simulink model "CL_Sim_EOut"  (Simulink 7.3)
settings: Solver=ode3  StartTime=0.0  StopTime=32  FixedStep=0.02  RelTol=1e-3
InitFcn:
  | [np,n]=size(time);
  | tfin= time(np);
  | Xini= xx(np,:);
  | Xfini= xfc(np,:);
  | dyin= dy(np,:);
  | dzin= dz(np,:);
  | Thin= Dthrust(np,:);
StopFcn:
  | Pl2
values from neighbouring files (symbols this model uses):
  Afc = [    [fcs.m]
  Bfc = [    [fcs.m]
  Cfc = [    [fcs.m]
  d2r = pi/180    (= 0.0174532925199)    [run.m]
  Dfc = [    [fcs.m]
  LBThrust = 0.96097e+6    (= 960970)    [run.m]
undefined symbols (not defined in the file or in its folder): Av2, Bv2, Cv2, Dv2, ThVC_eo

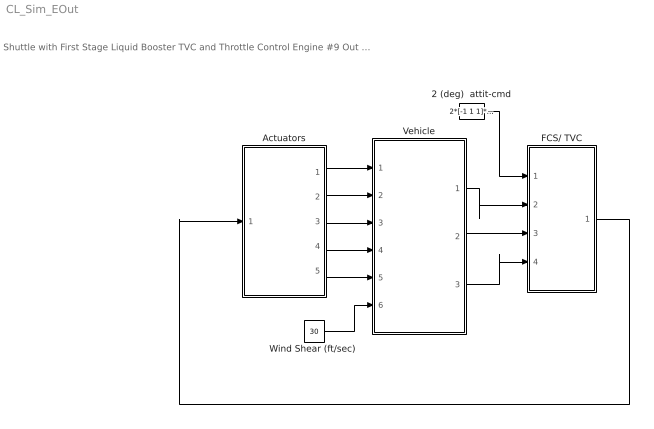
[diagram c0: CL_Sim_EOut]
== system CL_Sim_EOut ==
  note: Shuttle with First Stage Liquid Booster TVC and Throttle Control Engine #9 Out Simulation
  2 (deg)  attit-cmd : Constant  Value=2*[-1 1 1]*d2r  OutDataType=sfix(16)  OutScaling=2^0
  Actuators : Subsystem
  FCS/ TVC : Subsystem
  Vehicle : Subsystem
  "Wind Shear (ft/sec) " : Constant  Value=30  OutDataType=sfix(16)  OutScaling=2^0
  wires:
  FCS/ TVC/1(TVC) -> Actuators/1(TVC)
  Vehicle/1(atti) -> FCS/ TVC/2(atti)
  Vehicle/2(rate) -> FCS/ TVC/3(rate)
  Vehicle/3(accel) -> FCS/ TVC/4(accel)
  "Wind Shear (ft/sec) "/1 -> Vehicle/6(Gust)
  2 (deg)  attit-cmd/1 -> FCS/ TVC/1(atti-cmd)
  Actuators/1(dy (pitch)) -> Vehicle/1(dy)
  Actuators/5(DThrottle) -> Vehicle/5(Dthro)
  Actuators/4(dzdd) -> Vehicle/4(dzdd)
  Actuators/3(dz (yaw)) -> Vehicle/3(dz)
  Actuators/2(dydd) -> Vehicle/2(dydd)

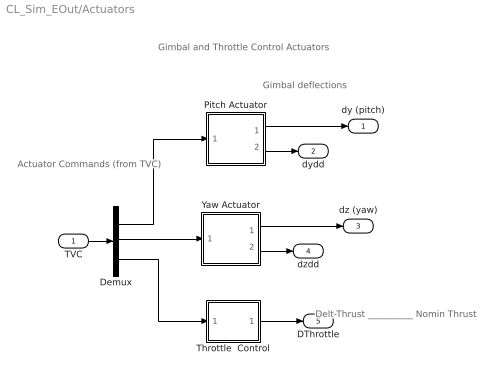
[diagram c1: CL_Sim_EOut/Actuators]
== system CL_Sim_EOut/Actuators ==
  note: Gimbal and Throttle Control Actuators
  note: Actuator Commands (from TVC)
  note: Gimbal deflections
  note: Delt-Thrust __________ Nomin Thrust
  TVC : Inport  OutDataType=sfix(16)  OutScaling=2^0
  Demux : Demux  Outputs=[9, 9, 6]
  Pitch Actuator : Subsystem
  Throttle  Control : Subsystem
  Yaw Actuator : Subsystem
  dy (pitch) : Outport  OutDataType=sfix(16)  OutScaling=2^0
  dydd : Outport  Port=2  OutDataType=sfix(16)  OutScaling=2^0
  dz (yaw) : Outport  Port=3  OutDataType=sfix(16)  OutScaling=2^0
  dzdd : Outport  Port=4  OutDataType=sfix(16)  OutScaling=2^0
  DThrottle : Outport  Port=5  OutDataType=sfix(16)  OutScaling=2^0
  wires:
  Demux/3 -> Throttle  Control/1(thi)
  Demux/1 -> Pitch Actuator/1(dy-c)
  Demux/2 -> Yaw Actuator/1(dz-c)
  Pitch Actuator/1(dy) -> dy (pitch)/1
  TVC/1 -> Demux/1
  Throttle  Control/1(tho) -> DThrottle/1
  Yaw Actuator/1(dz) -> dz (yaw)/1
  Pitch Actuator/2(dydd) -> dydd/1
  Yaw Actuator/2(dzdd) -> dzdd/1

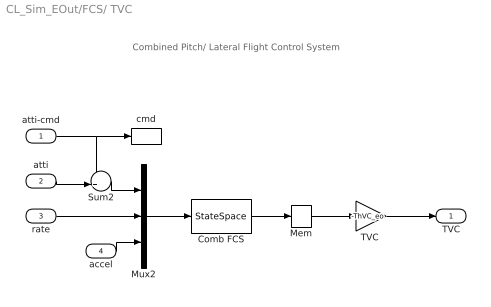
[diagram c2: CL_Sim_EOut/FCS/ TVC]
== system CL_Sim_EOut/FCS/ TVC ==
  note: Combined Pitch/ Lateral Flight Control System
  atti-cmd : Inport  OutDataType=sfix(16)  OutScaling=2^0
  atti : Inport  Port=2  OutDataType=sfix(16)  OutScaling=2^0
  rate : Inport  Port=3  OutDataType=sfix(16)  OutScaling=2^0
  accel : Inport  Port=4  OutDataType=sfix(16)  OutScaling=2^0
  Comb FCS : StateSpace  A=Afc  B=Bfc  C=Cfc  D=Dfc  X0=Xfini
  Mem : Memory
  Mux2 : Mux  Inputs=[3, 3, 2]
  Sum2 : Sum  Inputs=-+|  OutDataType=sfix(16)  OutScaling=2^0
  "TVC " : Gain  Gain=-ThVC_eo  Multiplication=Matrix(K*u) (u vector)  ParameterDataType=sfix(16)  ParameterScaling=2^0  OutDataType=sfix(16)  OutScaling=2^0
  cmd : ToWorkspace  VariableName=cmd2  SampleTime=-1  SaveFormat=Array
  TVC : Outport  OutDataType=sfix(16)  OutScaling=2^0
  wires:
  Mux2/1 -> Comb FCS/1
  accel/1 -> Mux2/3
  rate/1 -> Mux2/2
  "TVC "/1 -> TVC/1
  Sum2/1 -> Mux2/1
  atti/1 -> Sum2/2
  atti-cmd/1 -> Sum2/1, cmd/1
  Mem/1 -> "TVC "/1
  Comb FCS/1 -> Mem/1

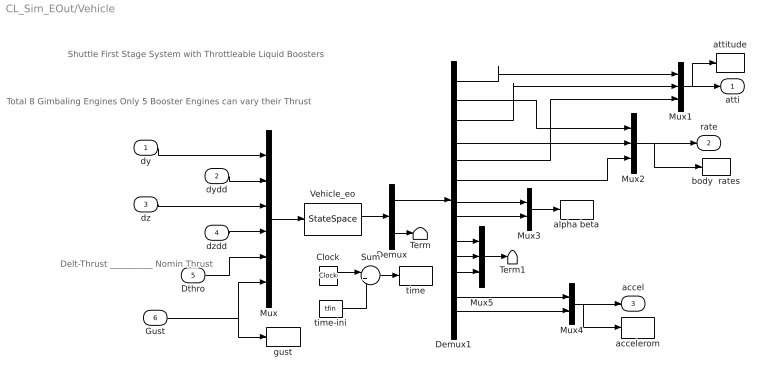
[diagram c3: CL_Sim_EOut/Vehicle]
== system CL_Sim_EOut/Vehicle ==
  note: Shuttle First Stage System with Throttleable Liquid Boosters
  note: Total 8 Gimbaling Engines Only 5 Booster Engines can vary their Thrust
  note: Delt-Thrust __________ Nomin Thrust
  dy : Inport  OutDataType=sfix(16)  OutScaling=2^0
  dydd : Inport  Port=2  OutDataType=sfix(16)  OutScaling=2^0
  dz : Inport  Port=3  OutDataType=sfix(16)  OutScaling=2^0
  dzdd : Inport  Port=4  OutDataType=sfix(16)  OutScaling=2^0
  Dthro : Inport  Port=5  OutDataType=sfix(16)  OutScaling=2^0
  Gust : Inport  Port=6  OutDataType=sfix(16)  OutScaling=2^0
  Clock : Clock
  Demux : Demux  Outputs=[13,18]
  Demux1 : Demux  Outputs=13
  Mux : Mux  Inputs=[9, 9, 9, 9, 6, 1]
  Mux1 : Mux  Inputs=3
  Mux2 : Mux  Inputs=3
  Mux3 : Mux  Inputs=2
  Mux4 : Mux  Inputs=2
  Mux5 : Mux  Inputs=3
  Sum : Sum  Inputs=|++  OutDataType=sfix(16)  OutScaling=2^0
  Term : Terminator
  Term1 : Terminator
  Vehicle_eo : StateSpace  A=Av2  B=Bv2  C=Cv2  D=Dv2  X0=Xini
  accelerom : ToWorkspace  VariableName=accel2  SampleTime=-1  SaveFormat=Array
  alpha beta : ToWorkspace  VariableName=albet2  SampleTime=-1  SaveFormat=Array
  attitude : ToWorkspace  VariableName=attit2  SampleTime=-1  SaveFormat=Array
  body  rates : ToWorkspace  VariableName=wb2  SampleTime=-1  SaveFormat=Array
  gust : ToWorkspace  VariableName=Gust2  SampleTime=-1  SaveFormat=Array
  time : ToWorkspace  VariableName=time2  SampleTime=-1  SaveFormat=Array
  time-ini : Constant  Value=tfin  OutDataType=sfix(16)  OutScaling=2^0
  atti : Outport  OutDataType=sfix(16)  OutScaling=2^0
  rate : Outport  Port=2  OutDataType=sfix(16)  OutScaling=2^0
  accel : Outport  Port=3  OutDataType=sfix(16)  OutScaling=2^0
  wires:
  Mux/1 -> Vehicle_eo/1
  Vehicle_eo/1 -> Demux/1
  Demux/1 -> Demux1/1
  Demux/2 -> Term/1
  Demux1/1 -> Mux1/1
  Demux1/3 -> Mux1/2
  Demux1/5 -> Mux1/3
  Demux1/2 -> Mux2/1
  Demux1/4 -> Mux2/2
  Demux1/6 -> Mux2/3
  Demux1/7 -> Mux3/1
  Demux1/8 -> Mux3/2
  Demux1/12 -> Mux4/1
  Demux1/13 -> Mux4/2
  Mux2/1 -> rate/1, body  rates/1
  Mux4/1 -> accel/1, accelerom/1
  dy/1 -> Mux/1
  dydd/1 -> Mux/2
  dz/1 -> Mux/3
  dzdd/1 -> Mux/4
  Demux1/9 -> Mux5/1
  Demux1/10 -> Mux5/2
  Demux1/11 -> Mux5/3
  Mux5/1 -> Term1/1
  Mux3/1 -> alpha beta/1
  Mux1/1 -> atti/1, attitude/1
  Gust/1 -> Mux/6, gust/1
  Clock/1 -> Sum/1
  Sum/1 -> time/1
  time-ini/1 -> Sum/2
  Dthro/1 -> Mux/5

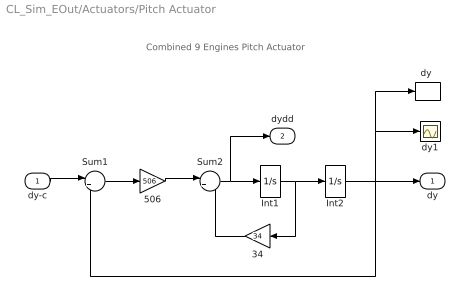
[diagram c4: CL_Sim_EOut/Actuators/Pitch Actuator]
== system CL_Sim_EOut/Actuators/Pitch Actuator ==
  note: Combined 9 Engines Pitch Actuator
  dy-c : Inport  PortDimensions=9  OutDataType=sfix(16)  OutScaling=2^0
  34 : Gain  Gain=34  ParameterDataType=sfix(16)  ParameterScaling=2^0  OutDataType=sfix(16)  OutScaling=2^0
  506 : Gain  Gain=506  ParameterDataType=sfix(16)  ParameterScaling=2^0  OutDataType=sfix(16)  OutScaling=2^0
  Int1 : Integrator
  Int2 : Integrator  InitialCondition=dyin
  Sum1 : Sum  Inputs=|+-  OutDataType=sfix(16)  OutScaling=2^0
  Sum2 : Sum  Inputs=|+-  OutDataType=sfix(16)  OutScaling=2^0
  "dy " : ToWorkspace  VariableName=dy2  SampleTime=-1  SaveFormat=Array
  dy1 : Scope
  dy : Outport  OutDataType=sfix(16)  OutScaling=2^0
  dydd : Outport  Port=2  OutDataType=sfix(16)  OutScaling=2^0
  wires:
  Sum2/1 -> Int1/1, dydd/1
  Int2/1 -> dy/1, dy1/1, "dy "/1, Sum1/2
  Int1/1 -> Int2/1, 34/1
  34/1 -> Sum2/2
  506/1 -> Sum2/1
  Sum1/1 -> 506/1
  dy-c/1 -> Sum1/1

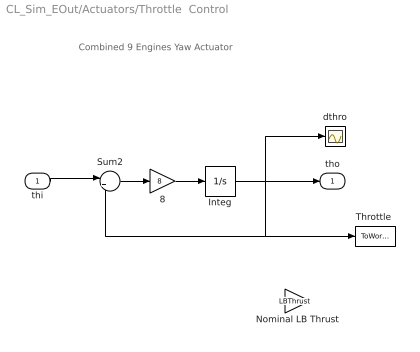
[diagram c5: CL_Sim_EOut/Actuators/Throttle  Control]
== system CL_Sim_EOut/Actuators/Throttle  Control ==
  note: Combined 9 Engines Yaw Actuator
  thi : Inport  PortDimensions=6  OutDataType=sfix(16)  OutScaling=2^0
  8 : Gain  Gain=8  ParameterDataType=sfix(16)  ParameterScaling=2^0  OutDataType=sfix(16)  OutScaling=2^0
  Integ : Integrator  InitialCondition=Thin
  Nominal LB Thrust : Gain  Gain=LBThrust  ParameterDataType=sfix(16)  ParameterScaling=2^0  OutDataType=sfix(16)  OutScaling=2^0
  Sum2 : Sum  Inputs=|+-  OutDataType=sfix(16)  OutScaling=2^0
  "Throttle " : ToWorkspace  VariableName=Dthrust2  SampleTime=-1  SaveFormat=Array
  dthro : Scope
  tho : Outport  OutDataType=sfix(16)  OutScaling=2^0
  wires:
  Sum2/1 -> 8/1
  8/1 -> Integ/1
  Integ/1 -> tho/1, dthro/1, Sum2/2, "Throttle "/1
  thi/1 -> Sum2/1

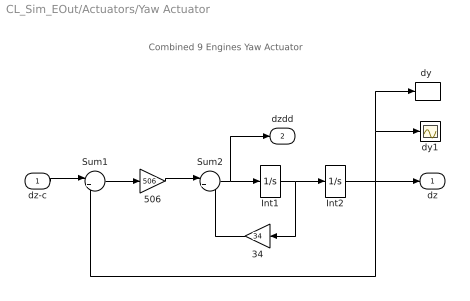
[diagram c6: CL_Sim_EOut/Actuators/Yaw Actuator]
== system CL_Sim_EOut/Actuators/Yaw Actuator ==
  note: Combined 9 Engines Yaw Actuator
  dz-c : Inport  PortDimensions=9  OutDataType=sfix(16)  OutScaling=2^0
  34 : Gain  Gain=34  ParameterDataType=sfix(16)  ParameterScaling=2^0  OutDataType=sfix(16)  OutScaling=2^0
  506 : Gain  Gain=506  ParameterDataType=sfix(16)  ParameterScaling=2^0  OutDataType=sfix(16)  OutScaling=2^0
  Int1 : Integrator
  Int2 : Integrator  InitialCondition=dzin
  Sum1 : Sum  Inputs=|+-  OutDataType=sfix(16)  OutScaling=2^0
  Sum2 : Sum  Inputs=|+-  OutDataType=sfix(16)  OutScaling=2^0
  "dy " : ToWorkspace  VariableName=dz2  SampleTime=-1  SaveFormat=Array
  dy1 : Scope
  dz : Outport  OutDataType=sfix(16)  OutScaling=2^0
  dzdd : Outport  Port=2  OutDataType=sfix(16)  OutScaling=2^0
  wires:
  Sum2/1 -> Int1/1, dzdd/1
  Int2/1 -> dz/1, dy1/1, "dy "/1, Sum1/2
  Int1/1 -> Int2/1, 34/1
  34/1 -> Sum2/2
  506/1 -> Sum2/1
  Sum1/1 -> 506/1
  dz-c/1 -> Sum1/1
